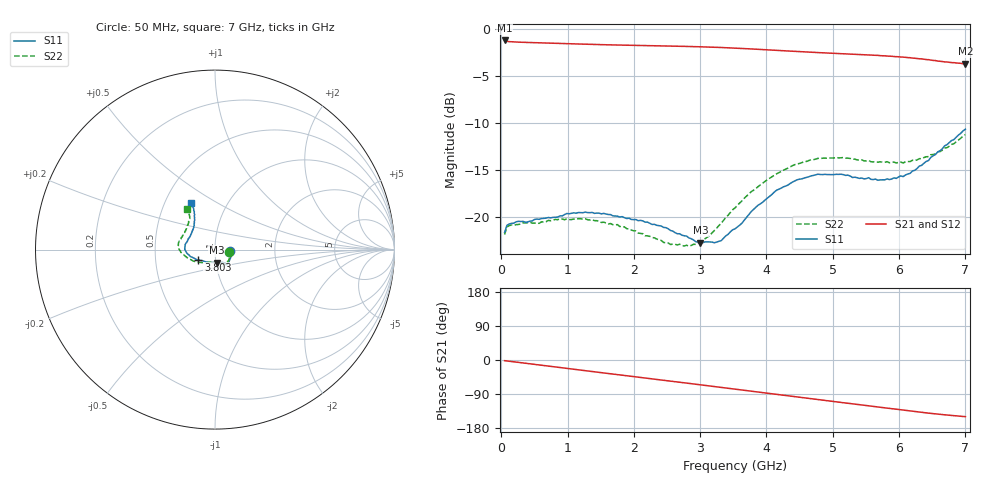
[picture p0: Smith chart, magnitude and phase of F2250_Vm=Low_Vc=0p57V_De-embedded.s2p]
! Integrated Device Technology
! Corporate Headquarters
! 6024 Silver Creek Valley Road
! San Jose, CA 95138  USA
! Phone:  1-408-284-8200
! Toll Free:  1-800-223-1366
! Webpage:  http://www.idt.com/
! Timing and RF Division
! 515 Groton Road, Suite 102
! Westford, MA 01886-6024
! Device:  F2250
! Description: Voltage Variable RF Attenuator
! Frequency:  50.0 -  6000.00 MHz
! Package:  3x3 mm Thin QFN Plastic Package: 16 pin
! Ports:  2 RF, 3 DC
!  Pin  1  = GND
!  Pin  2  = NC
!  Pin  3  = RF1  = Port 1
!  Pin  4  = NC
!  Pin  5  = GND
!  Pin  6  = GND
!  Pin  7  = GND
!  Pin  8  = GND
!  Pin  9  = NC
!  Pin 10  = RF2  = Port 2
!  Pin 11  = NC
!  Pin 12  = GND
!  Pin 13  = GND
!  Pin 14  = VCNTRL
!  Pin 15  = VDD
!  Pin 16  = VMODE
! Vcntrl:  0.570 Volts
! Vmode:  +0.000 Volts
! Vdd:  +3.30  Volts
! Current:  1.134 mA
! Data:  The device was measured on a the F2250 evaluation board which has
!  individual transmission lines to the RF pins.  Data was collected
!  using a calibrated network analyzer.  The evaluation board was
!  de-embedded using a TRL calibration technique.
!  The reference plane is the edge of the package pin.
! Misc:  SN 10
!  Action Tracker AT0258
! Date Measured:  2014-11-26
! Date:  2015-10-15  MJV
! Note:
!  Integrated Device Technology supplies this data as a sample of measured
!  data at the package pin for this product.  Your particular data for this
!  product may vary.
!  Data was taken at 25 degrees C.
!  Integrated Device Technology reserves the right to change this data at anytime.
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# GHz S dB R 50
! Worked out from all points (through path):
!   201 points, 50 MHz to 7 GHz, reference 50 ohm
!   highest |S21| = -1.19 dB at 50 MHz (marker M1); lowest = -3.7 dB at 7 GHz (marker M2)
!   group delay of S21, straight-line fit = 60.1 ps
!   lowest |S11| = -22.8 dB at 3.004 GHz (marker M3), VSWR 1.16, Z = 50.5 - j7.31 ohm
!   |S11| at or under -10 dB: start of sweep to end of sweep
!   |S22| runs from -23.1 to -11.2 dB; largest |S21 - S12| = 0.00042
!   S11 on the Smith chart (normalised r, x): 50 MHz: 1.18, -0.02; 3.803 GHz: 0.83, -0.10; 7 GHz: 0.68, +0.39
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0.05  -21.67 -6.7  -1.19 -1.8  -1.19 -1.8  -21.89 -7.7
0.08475  -20.90 -6.7  -1.28 -2.5  -1.28 -2.5  -21.08 -7.3
0.15425  -20.69 -8.8  -1.33 -4.0  -1.33 -4.0  -20.87 -9.1
0.6755  -20.14 -28.7  -1.46 -15.4  -1.46 -15.4  -20.52 -31.9
1.2315  -19.56 -46.0  -1.58 -27.4  -1.58 -27.4  -20.25 -53.6
1.75275  -19.93 -52.8  -1.68 -38.5  -1.68 -38.5  -20.83 -63.1
2.37825  -20.94 -55.3  -1.77 -51.8  -1.77 -51.8  -22.46 -71.1
2.552  -21.46 -58.6  -1.79 -55.6  -1.79 -55.6  -22.96 -76.9
2.83  -22.25 -69.4  -1.84 -61.7  -1.83 -61.7  -23.13 -92.7
3.00375  -22.77 -82.2  -1.87 -65.6  -1.86 -65.6  -22.61 -105.6
3.14275  -22.68 -93.1  -1.90 -68.6  -1.90 -68.6  -22.02 -116.7
3.3165  -22.54 -110.9  -1.94 -72.5  -1.94 -72.5  -20.69 -128.4
3.525  -21.28 -129.0  -2.01 -77.2  -2.00 -77.2  -19.05 -140.6
3.803  -19.22 -147.8  -2.11 -83.3  -2.11 -83.4  -17.16 -153.4
4.1505  -17.17 -162.8  -2.25 -91.0  -2.25 -91.0  -15.42 -167.4
4.7065  -15.59 -179.0  -2.46 -103.0  -2.46 -103.0  -13.91 178.4
5.15825  -15.50 169.9  -2.62 -112.7  -2.62 -112.7  -13.67 168.7
5.85325  -16.02 146.2  -2.87 -127.6  -2.87 -127.6  -14.23 152.9
6.166  -15.36 134.0  -3.03 -134.4  -3.03 -134.4  -14.10 143.8
6.444  -13.99 124.4  -3.24 -140.2  -3.24 -140.2  -13.58 134.3
6.82625  -11.77 117.5  -3.56 -146.9  -3.56 -146.9  -12.21 126.1
7  -10.66 116.6  -3.68 -149.6  -3.68 -149.6  -11.23 124.6
